(* Logix 5000 AddOnInstructionDefinition export Banner_QCM50_Param_v4; software revision 33.00; part 2 of 2 *)
(* tags used below, declared in another part *)
   QCM50 : Banner_QCM50_v4;
   Port_Data : Banner_IOL_Port_v4;
   Port : INT;   // Enter the Port number that this AOI is to work with.
   K : SINT;   // 1,3,or 5. Based off number after the K in part number.
   Local_Control : DINT;
   Command_Being_Processed : BOOL;
   Update_Archive : BOOL;
   Index_Write_Inprocess : DINT;
   Index_Write_Control : DINT;
   Inprocess_Index : DINT;
   CWC3_Index : SINT;
   CWC2_Index : SINT;
   CWC1_Index : SINT;
   C_Limit : SINT[2];
   CW_Index : SINT;
(* Banner_QCM50_Param_v4, continued *)

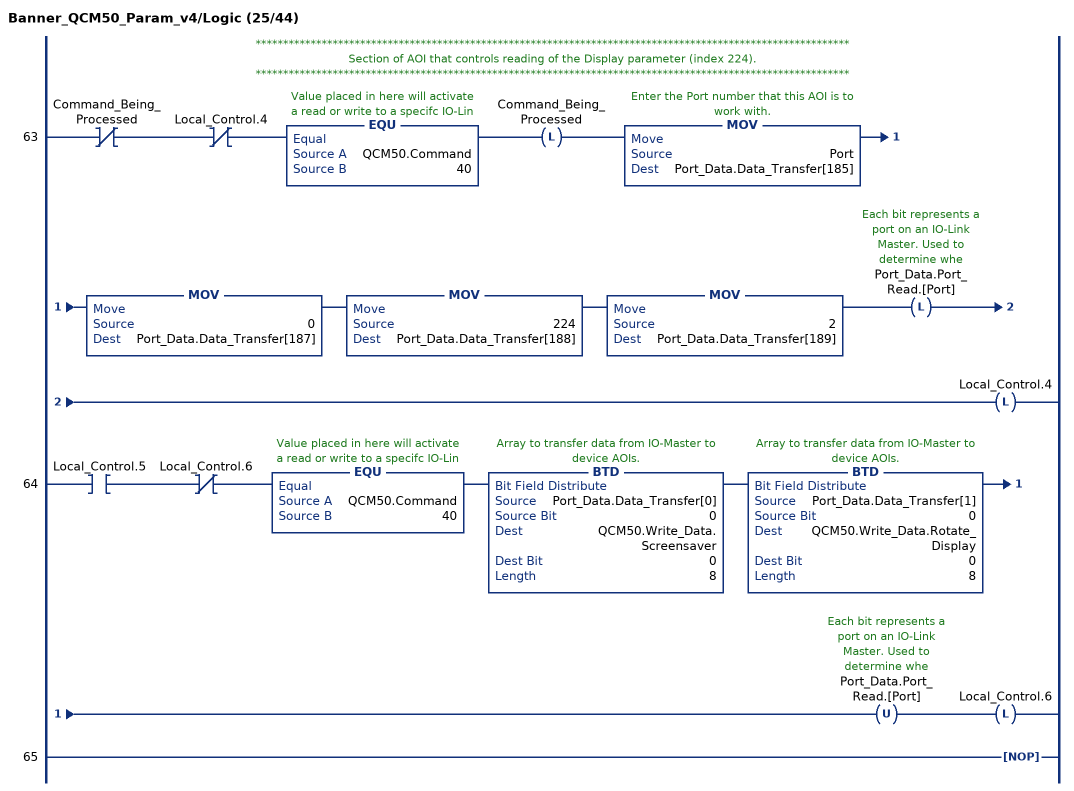
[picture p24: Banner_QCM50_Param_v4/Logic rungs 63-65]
   // ************************************************************************************************************
   // Section of AOI that controls reading of the Display parameter (index 224).
   // ************************************************************************************************************
   63: XIO(Command_Being_Processed)XIO(Local_Control.4)EQU(QCM50.Command,40)OTL(Command_Being_Processed)MOV(Port,Port_Data.Data_Transfer[185])MOV(0,Port_Data.Data_Transfer[187])MOV(224,Port_Data.Data_Transfer[188])MOV(2,Port_Data.Data_Transfer[189])OTL(Port_Data.Port_Read.[Port])OTL(Local_Control.4);
   64: XIC(Local_Control.5)XIO(Local_Control.6)EQU(QCM50.Command,40)BTD(Port_Data.Data_Transfer[0],0,QCM50.Write_Data.Screensaver,0,8)BTD(Port_Data.Data_Transfer[1],0,QCM50.Write_Data.Rotate_Display,0,8)OTU(Port_Data.Port_Read.[Port])OTL(Local_Control.6);
   65: NOP();
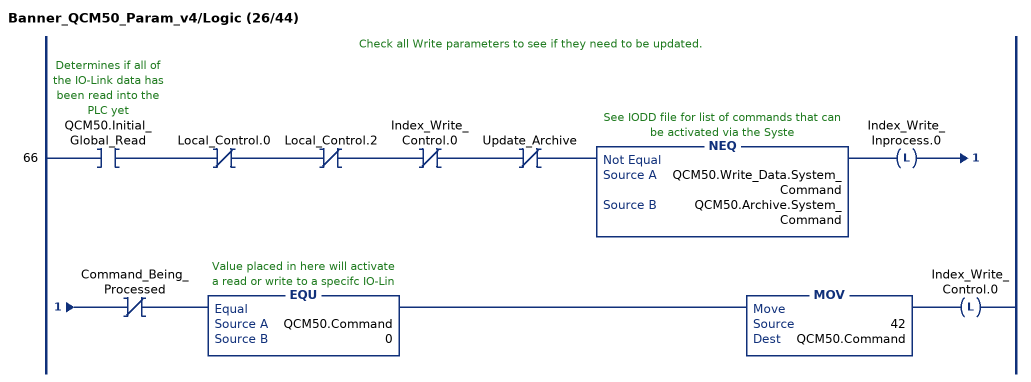
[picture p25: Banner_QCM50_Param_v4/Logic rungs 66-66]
   // Check all Write parameters to see if they need to be updated.
   66: XIC(QCM50.Initial_Global_Read)XIO(Local_Control.0)XIO(Local_Control.2)XIO(Index_Write_Control.0)XIO(Update_Archive)NEQ(QCM50.Write_Data.System_Command,QCM50.Archive.System_Command)OTL(Index_Write_Inprocess.0)XIO(Command_Being_Processed)EQU(QCM50.Command,0)MOV(42,QCM50.Command)OTL(Index_Write_Control.0);
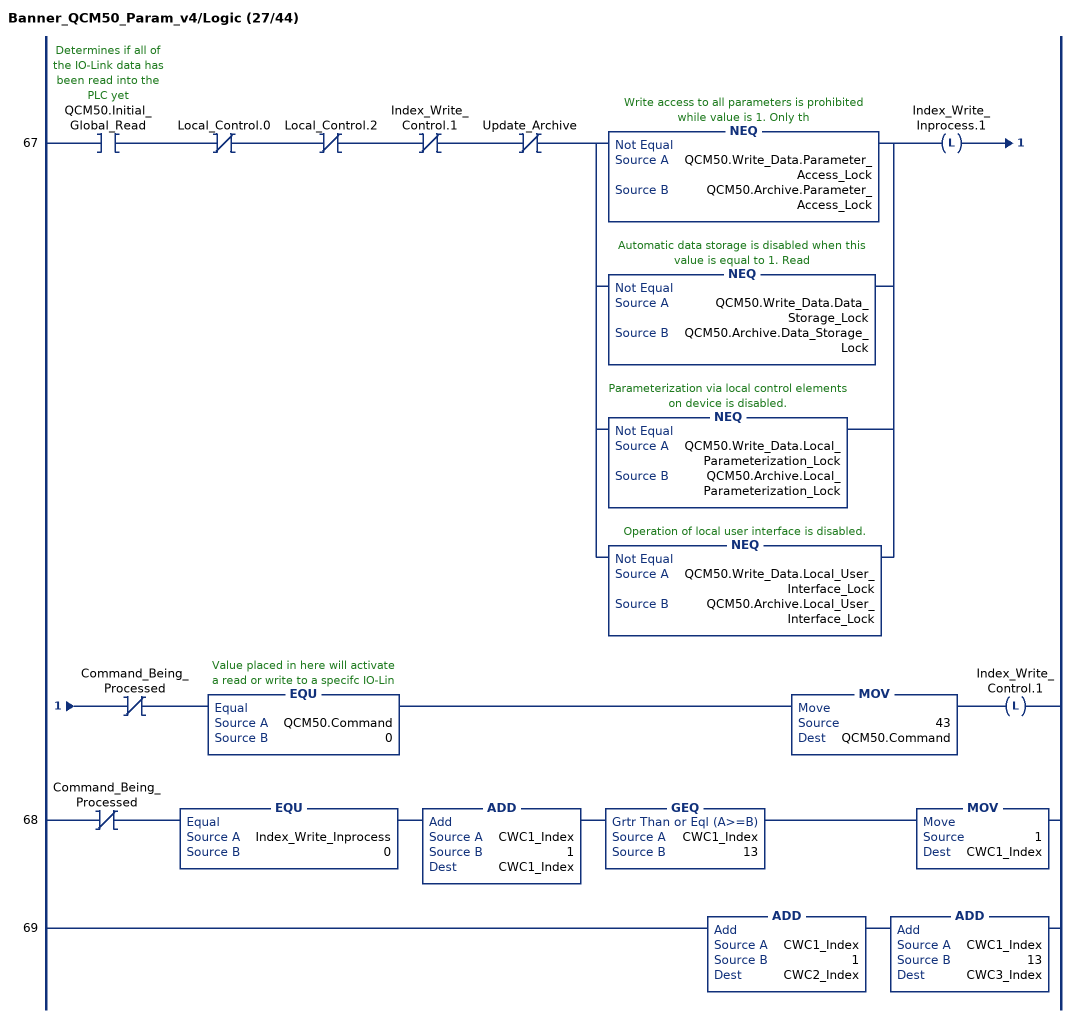
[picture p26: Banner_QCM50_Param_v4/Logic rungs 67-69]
   67: XIC(QCM50.Initial_Global_Read)XIO(Local_Control.0)XIO(Local_Control.2)XIO(Index_Write_Control.1)XIO(Update_Archive)[NEQ(QCM50.Write_Data.Parameter_Access_Lock,QCM50.Archive.Parameter_Access_Lock) ,NEQ(QCM50.Write_Data.Data_Storage_Lock,QCM50.Archive.Data_Storage_Lock) ,NEQ(QCM50.Write_Data.Local_Parameterization_Lock,QCM50.Archive.Local_Parameterization_Lock) ,NEQ(QCM50.Write_Data.Local_User_Interface_Lock,QCM50.Archive.Local_User_Interface_Lock) ]OTL(Index_Write_Inprocess.1)XIO(Command_Being_Processed)EQU(QCM50.Command,0)MOV(43,QCM50.Command)OTL(Index_Write_Control.1);
   68: XIO(Command_Being_Processed)EQU(Index_Write_Inprocess,0)ADD(CWC1_Index,1,CWC1_Index)GEQ(CWC1_Index,13)MOV(1,CWC1_Index);
   69: ADD(CWC1_Index,1,CWC2_Index)ADD(CWC1_Index,13,CWC3_Index);
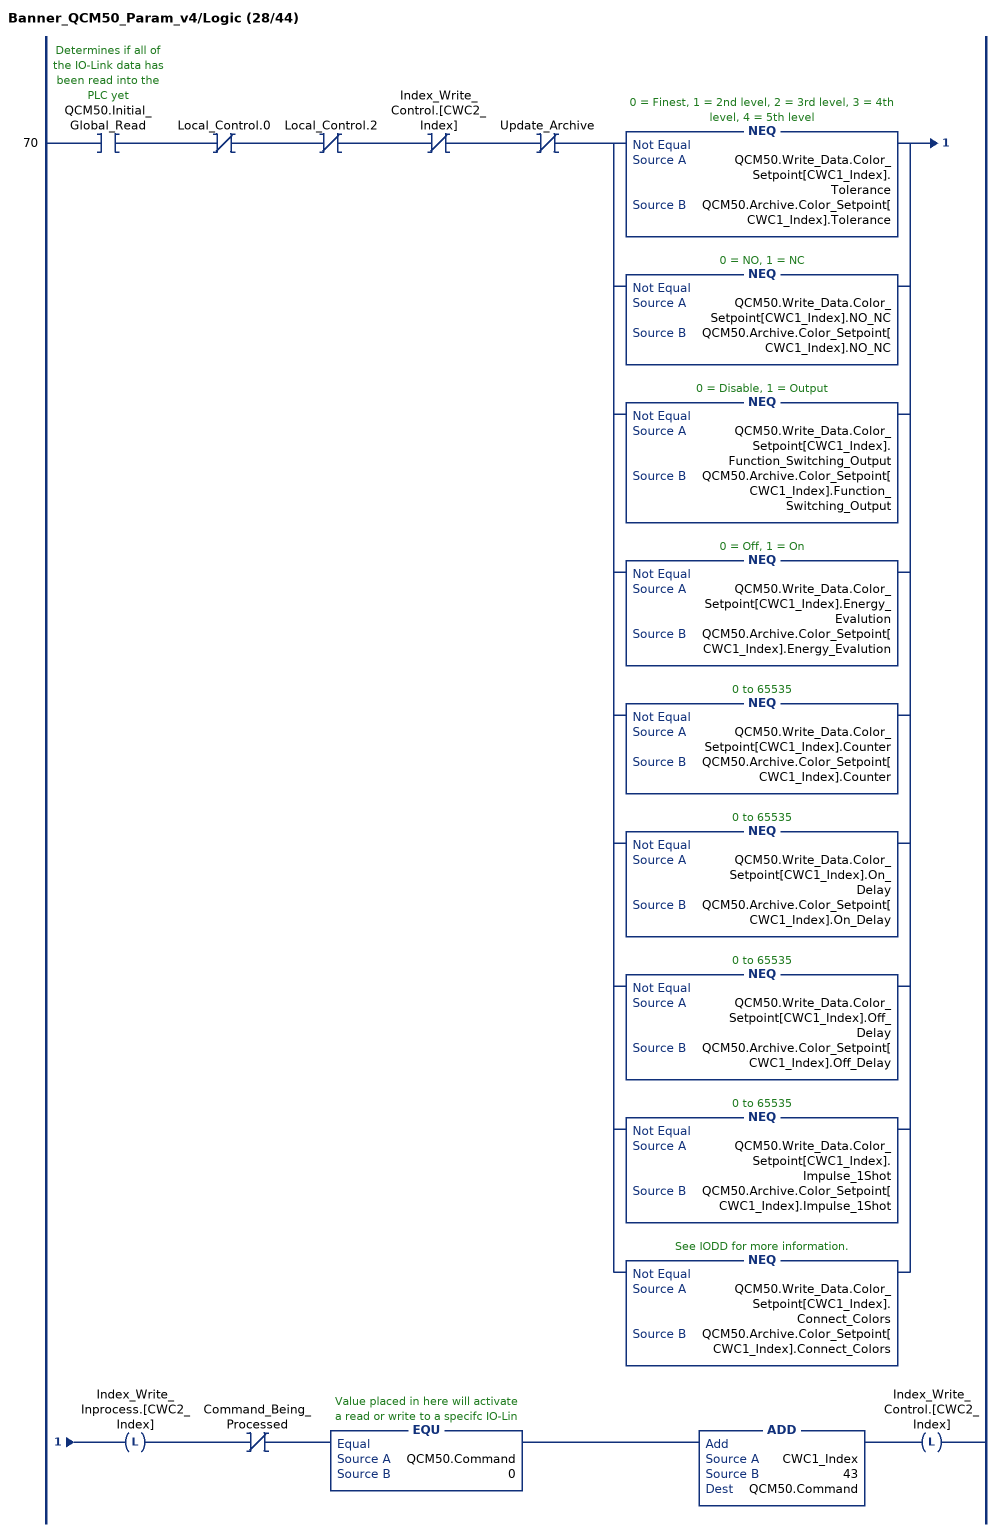
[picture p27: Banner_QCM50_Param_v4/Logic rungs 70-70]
   70: XIC(QCM50.Initial_Global_Read)XIO(Local_Control.0)XIO(Local_Control.2)XIO(Index_Write_Control.[CWC2_Index])XIO(Update_Archive)[NEQ(QCM50.Write_Data.Color_Setpoint[CWC1_Index].Tolerance,QCM50.Archive.Color_Setpoint[CWC1_Index].Tolerance) ,NEQ(QCM50.Write_Data.Color_Setpoint[CWC1_Index].NO_NC,QCM50.Archive.Color_Setpoint[CWC1_Index].NO_NC) ,NEQ(QCM50.Write_Data.Color_Setpoint[CWC1_Index].Function_Switching_Output,QCM50.Archive.Color_Setpoint[CWC1_Index].Function_Switching_Output) ,NEQ(QCM50.Write_Data.Color_Setpoint[CWC1_Index].Energy_Evalution,QCM50.Archive.Color_Setpoint[CWC1_Index].Energy_Evalution) ,NEQ(QCM50.Write_Data.Color_Setpoint[CWC1_Index].Counter,QCM50.Archive.Color_Setpoint[CWC1_Index].Counter) ,NEQ(QCM50.Write_Data.Color_Setpoint[CWC1_Index].On_Delay,QCM50.Archive.Color_Setpoint[CWC1_Index].On_Delay) ,NEQ(QCM50.Write_Data.Color_Setpoint[CWC1_Index].Off_Delay,QCM50.Archive.Color_Setpoint[CWC1_Index].Off_Delay) ,NEQ(QCM50.Write_Data.Color_Setpoint[CWC1_Index].Impulse_1Shot,QCM50.Archive.Color_Setpoint[CWC1_Index].Impulse_1Shot) ,NEQ(QCM50.Write_Data.Color_Setpoint[CWC1_Index].Connect_Colors,QCM50.Archive.Color_Setpoint[CWC1_Index].Connect_Colors) ]OTL(Index_Write_Inprocess.[CWC2_Index])XIO(Command_Being_Processed)EQU(QCM50.Command,0)ADD(CWC1_Index,43,QCM50.Command)OTL(Index_Write_Control.[CWC2_Index]);
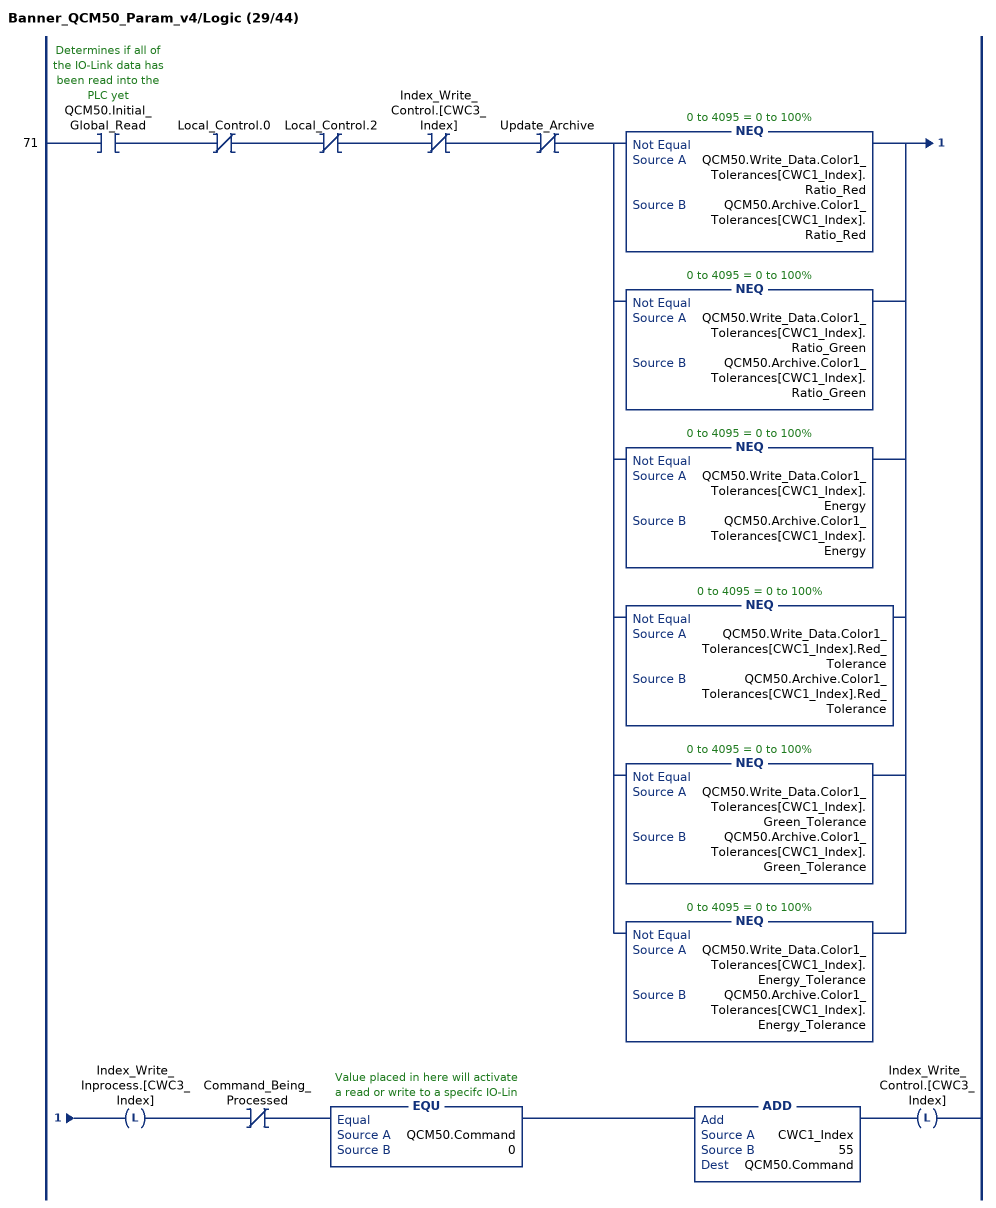
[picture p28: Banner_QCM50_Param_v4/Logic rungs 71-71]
   71: XIC(QCM50.Initial_Global_Read)XIO(Local_Control.0)XIO(Local_Control.2)XIO(Index_Write_Control.[CWC3_Index])XIO(Update_Archive)[NEQ(QCM50.Write_Data.Color1_Tolerances[CWC1_Index].Ratio_Red,QCM50.Archive.Color1_Tolerances[CWC1_Index].Ratio_Red) ,NEQ(QCM50.Write_Data.Color1_Tolerances[CWC1_Index].Ratio_Green,QCM50.Archive.Color1_Tolerances[CWC1_Index].Ratio_Green) ,NEQ(QCM50.Write_Data.Color1_Tolerances[CWC1_Index].Energy,QCM50.Archive.Color1_Tolerances[CWC1_Index].Energy) ,NEQ(QCM50.Write_Data.Color1_Tolerances[CWC1_Index].Red_Tolerance,QCM50.Archive.Color1_Tolerances[CWC1_Index].Red_Tolerance) ,NEQ(QCM50.Write_Data.Color1_Tolerances[CWC1_Index].Green_Tolerance,QCM50.Archive.Color1_Tolerances[CWC1_Index].Green_Tolerance) ,NEQ(QCM50.Write_Data.Color1_Tolerances[CWC1_Index].Energy_Tolerance,QCM50.Archive.Color1_Tolerances[CWC1_Index].Energy_Tolerance) ]OTL(Index_Write_Inprocess.[CWC3_Index])XIO(Command_Being_Processed)EQU(QCM50.Command,0)ADD(CWC1_Index,55,QCM50.Command)OTL(Index_Write_Control.[CWC3_Index]);
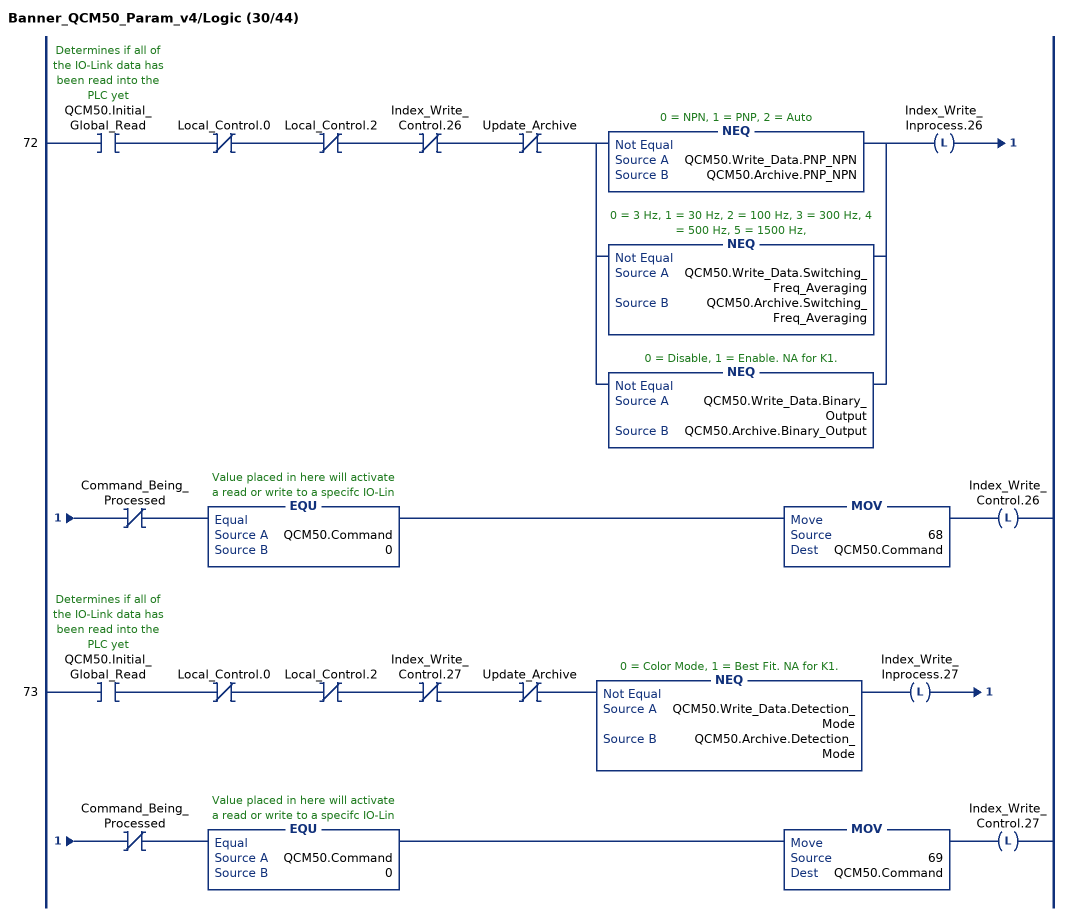
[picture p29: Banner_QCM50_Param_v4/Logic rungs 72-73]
   72: XIC(QCM50.Initial_Global_Read)XIO(Local_Control.0)XIO(Local_Control.2)XIO(Index_Write_Control.26)XIO(Update_Archive)[NEQ(QCM50.Write_Data.PNP_NPN,QCM50.Archive.PNP_NPN) ,NEQ(QCM50.Write_Data.Switching_Freq_Averaging,QCM50.Archive.Switching_Freq_Averaging) ,NEQ(QCM50.Write_Data.Binary_Output,QCM50.Archive.Binary_Output) ]OTL(Index_Write_Inprocess.26)XIO(Command_Being_Processed)EQU(QCM50.Command,0)MOV(68,QCM50.Command)OTL(Index_Write_Control.26);
   73: XIC(QCM50.Initial_Global_Read)XIO(Local_Control.0)XIO(Local_Control.2)XIO(Index_Write_Control.27)XIO(Update_Archive)NEQ(QCM50.Write_Data.Detection_Mode,QCM50.Archive.Detection_Mode)OTL(Index_Write_Inprocess.27)XIO(Command_Being_Processed)EQU(QCM50.Command,0)MOV(69,QCM50.Command)OTL(Index_Write_Control.27);
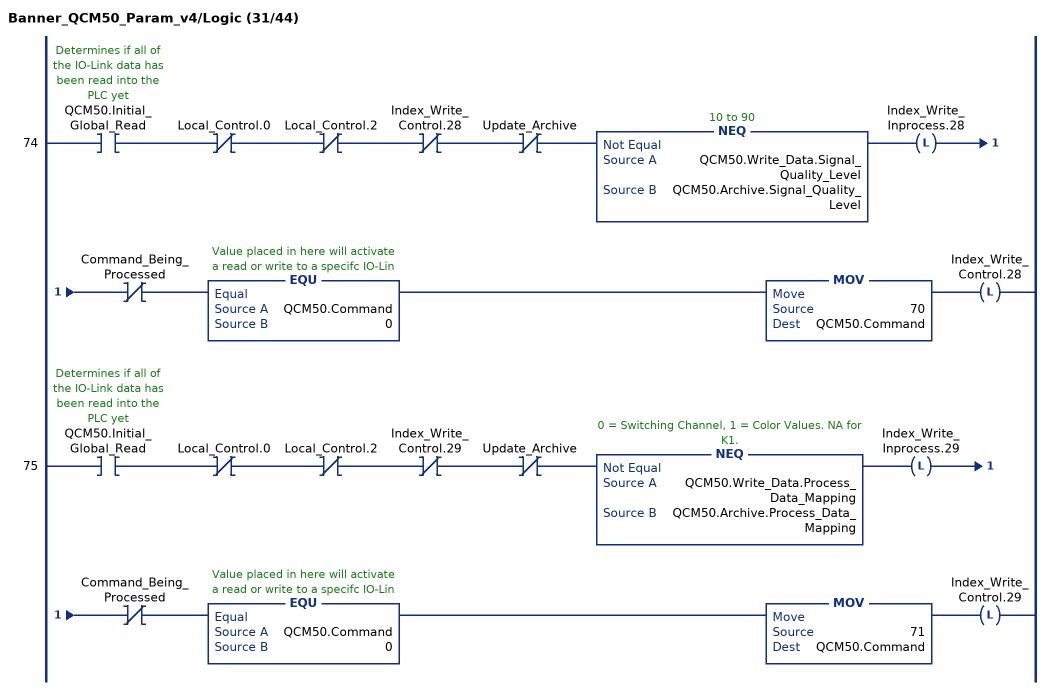
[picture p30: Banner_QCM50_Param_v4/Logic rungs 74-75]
   74: XIC(QCM50.Initial_Global_Read)XIO(Local_Control.0)XIO(Local_Control.2)XIO(Index_Write_Control.28)XIO(Update_Archive)NEQ(QCM50.Write_Data.Signal_Quality_Level,QCM50.Archive.Signal_Quality_Level)OTL(Index_Write_Inprocess.28)XIO(Command_Being_Processed)EQU(QCM50.Command,0)MOV(70,QCM50.Command)OTL(Index_Write_Control.28);
   75: XIC(QCM50.Initial_Global_Read)XIO(Local_Control.0)XIO(Local_Control.2)XIO(Index_Write_Control.29)XIO(Update_Archive)NEQ(QCM50.Write_Data.Process_Data_Mapping,QCM50.Archive.Process_Data_Mapping)OTL(Index_Write_Inprocess.29)XIO(Command_Being_Processed)EQU(QCM50.Command,0)MOV(71,QCM50.Command)OTL(Index_Write_Control.29);
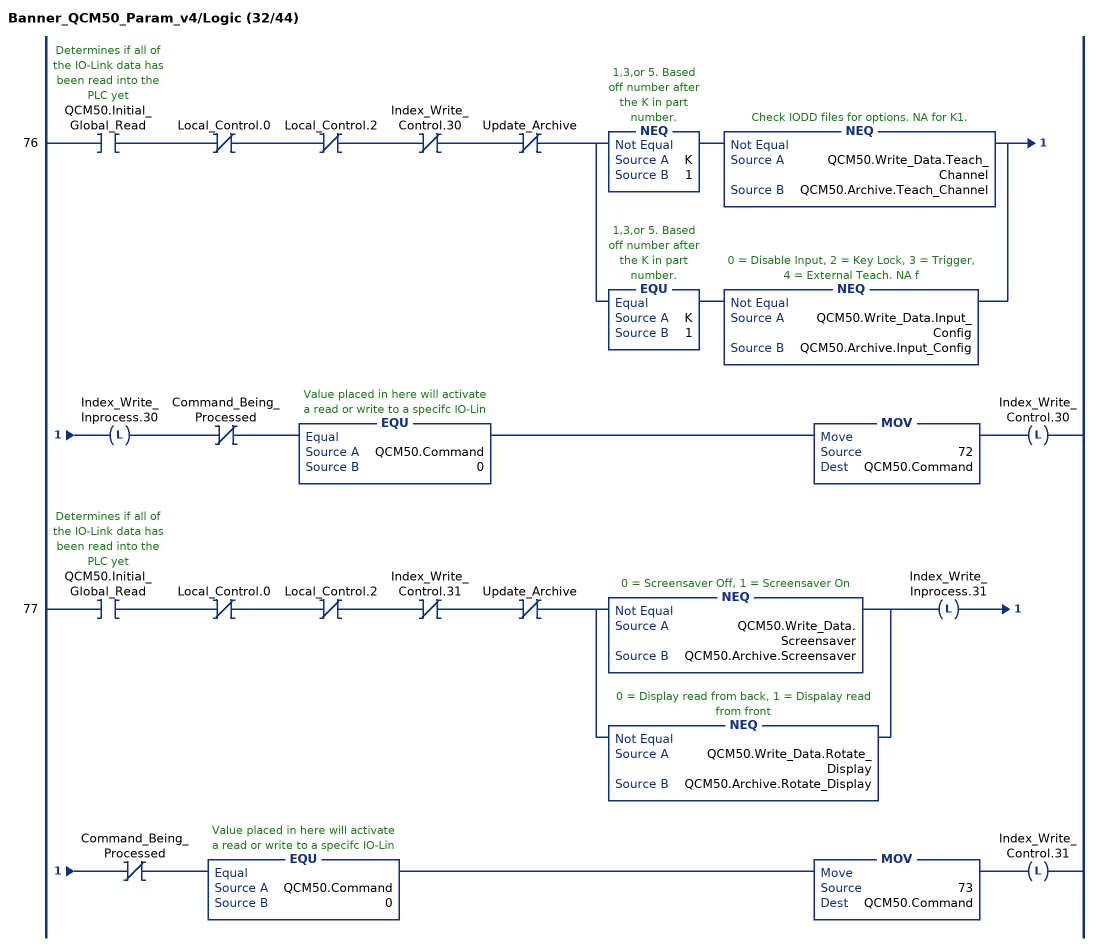
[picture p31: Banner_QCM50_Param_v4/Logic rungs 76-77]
   76: XIC(QCM50.Initial_Global_Read)XIO(Local_Control.0)XIO(Local_Control.2)XIO(Index_Write_Control.30)XIO(Update_Archive)[NEQ(K,1) NEQ(QCM50.Write_Data.Teach_Channel,QCM50.Archive.Teach_Channel) ,EQU(K,1) NEQ(QCM50.Write_Data.Input_Config,QCM50.Archive.Input_Config) ]OTL(Index_Write_Inprocess.30)XIO(Command_Being_Processed)EQU(QCM50.Command,0)MOV(72,QCM50.Command)OTL(Index_Write_Control.30);
   77: XIC(QCM50.Initial_Global_Read)XIO(Local_Control.0)XIO(Local_Control.2)XIO(Index_Write_Control.31)XIO(Update_Archive)[NEQ(QCM50.Write_Data.Screensaver,QCM50.Archive.Screensaver) ,NEQ(QCM50.Write_Data.Rotate_Display,QCM50.Archive.Rotate_Display) ]OTL(Index_Write_Inprocess.31)XIO(Command_Being_Processed)EQU(QCM50.Command,0)MOV(73,QCM50.Command)OTL(Index_Write_Control.31);
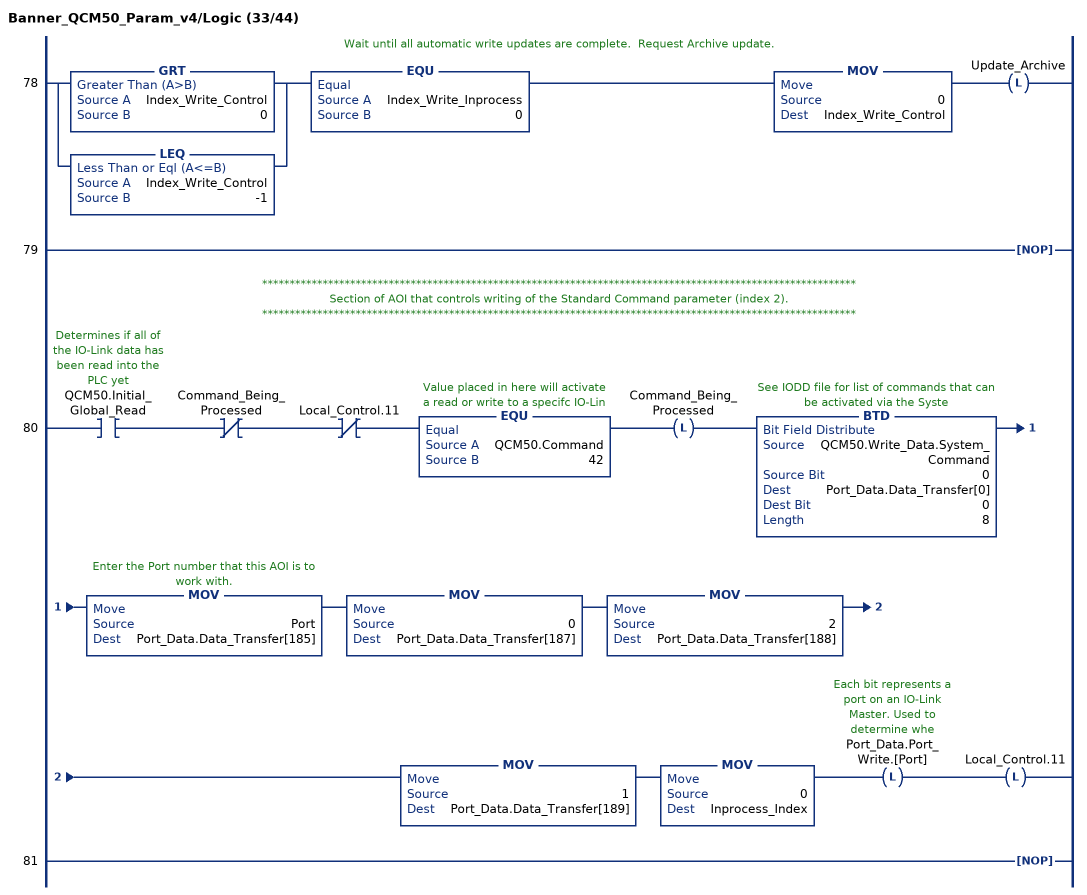
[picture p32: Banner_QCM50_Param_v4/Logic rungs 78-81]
   // Wait until all automatic write updates are complete.  Request Archive update.
   78: [GRT(Index_Write_Control,0) ,LEQ(Index_Write_Control,-1) ]EQU(Index_Write_Inprocess,0)MOV(0,Index_Write_Control)OTL(Update_Archive);
   79: NOP();
   // ************************************************************************************************************
   // Section of AOI that controls writing of the Standard Command parameter (index 2).
   // ************************************************************************************************************
   80: XIC(QCM50.Initial_Global_Read)XIO(Command_Being_Processed)XIO(Local_Control.11)EQU(QCM50.Command,42)OTL(Command_Being_Processed)BTD(QCM50.Write_Data.System_Command,0,Port_Data.Data_Transfer[0],0,8)MOV(Port,Port_Data.Data_Transfer[185])MOV(0,Port_Data.Data_Transfer[187])MOV(2,Port_Data.Data_Transfer[188])MOV(1,Port_Data.Data_Transfer[189])MOV(0,Inprocess_Index)OTL(Port_Data.Port_Write.[Port])OTL(Local_Control.11);
   81: NOP();
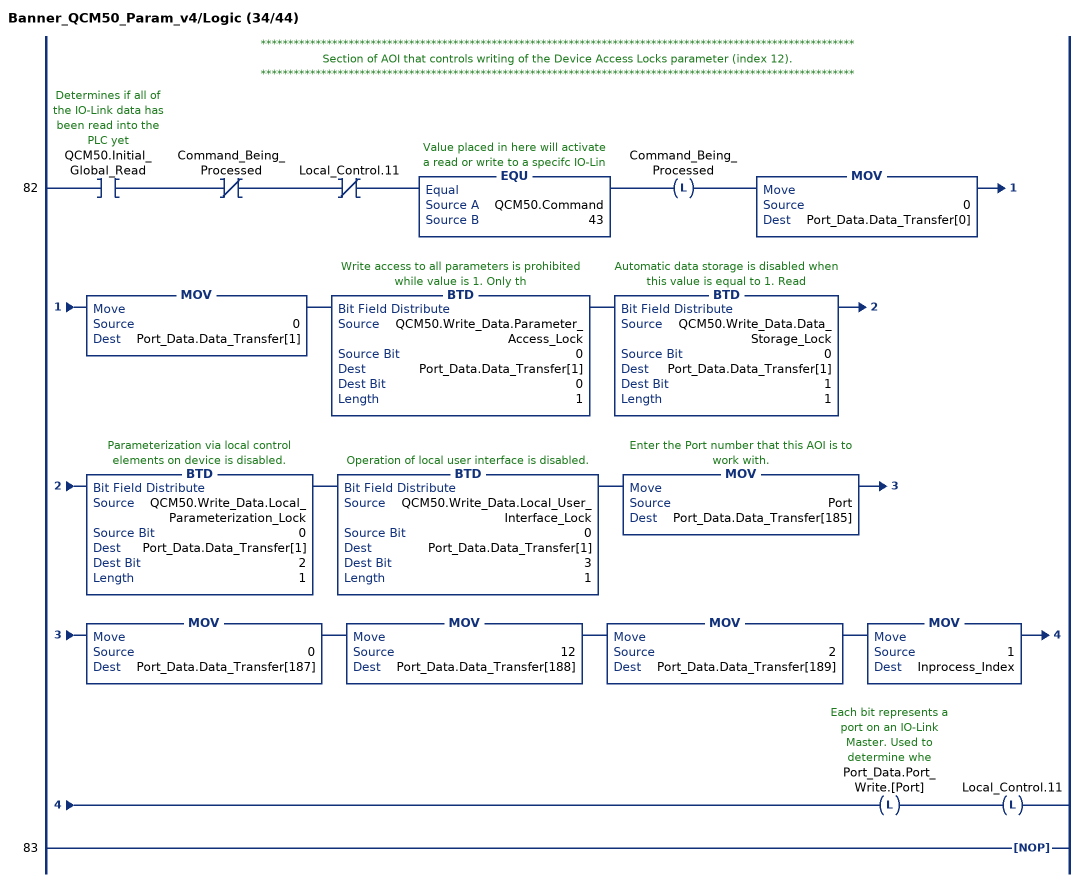
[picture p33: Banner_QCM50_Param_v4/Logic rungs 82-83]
   // ************************************************************************************************************
   // Section of AOI that controls writing of the Device Access Locks parameter (index 12).
   // ************************************************************************************************************
   82: XIC(QCM50.Initial_Global_Read)XIO(Command_Being_Processed)XIO(Local_Control.11)EQU(QCM50.Command,43)OTL(Command_Being_Processed)MOV(0,Port_Data.Data_Transfer[0])MOV(0,Port_Data.Data_Transfer[1])BTD(QCM50.Write_Data.Parameter_Access_Lock,0,Port_Data.Data_Transfer[1],0,1)BTD(QCM50.Write_Data.Data_Storage_Lock,0,Port_Data.Data_Transfer[1],1,1)BTD(QCM50.Write_Data.Local_Parameterization_Lock,0,Port_Data.Data_Transfer[1],2,1)BTD(QCM50.Write_Data.Local_User_Interface_Lock,0,Port_Data.Data_Transfer[1],3,1)MOV(Port,Port_Data.Data_Transfer[185])MOV(0,Port_Data.Data_Transfer[187])MOV(12,Port_Data.Data_Transfer[188])MOV(2,Port_Data.Data_Transfer[189])MOV(1,Inprocess_Index)OTL(Port_Data.Port_Write.[Port])OTL(Local_Control.11);
   83: NOP();
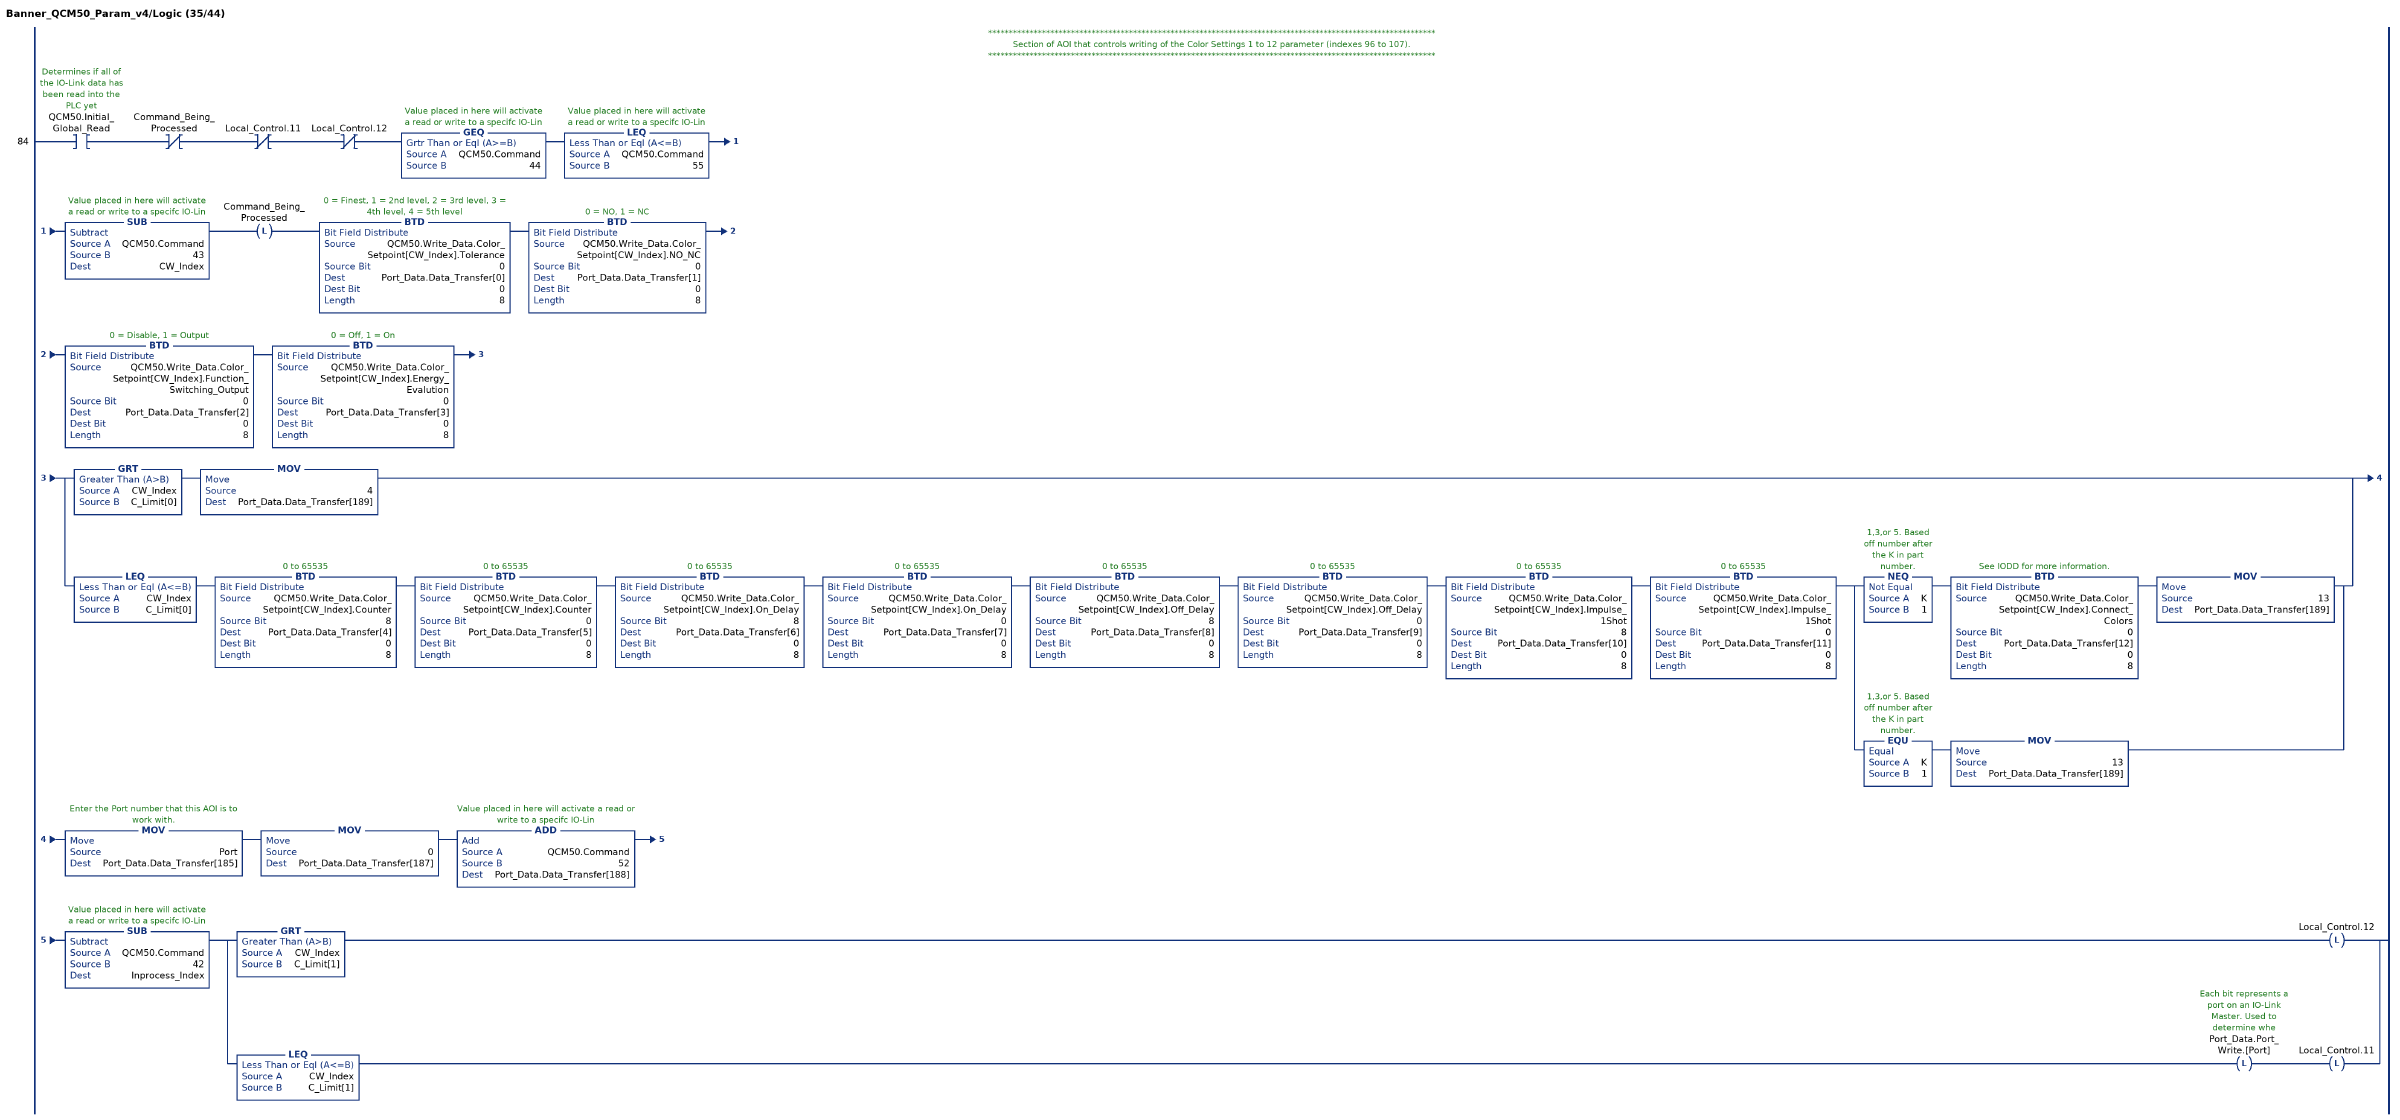
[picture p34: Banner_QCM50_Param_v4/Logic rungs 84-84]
   // ************************************************************************************************************
   // Section of AOI that controls writing of the Color Settings 1 to 12 parameter (indexes 96 to 107).
   // ************************************************************************************************************
   84: XIC(QCM50.Initial_Global_Read)XIO(Command_Being_Processed)XIO(Local_Control.11)XIO(Local_Control.12)GEQ(QCM50.Command,44)LEQ(QCM50.Command,55)SUB(QCM50.Command,43,CW_Index)OTL(Command_Being_Processed)BTD(QCM50.Write_Data.Color_Setpoint[CW_Index].Tolerance,0,Port_Data.Data_Transfer[0],0,8)BTD(QCM50.Write_Data.Color_Setpoint[CW_Index].NO_NC,0,Port_Data.Data_Transfer[1],0,8)BTD(QCM50.Write_Data.Color_Setpoint[CW_Index].Function_Switching_Output,0,Port_Data.Data_Transfer[2],0,8)BTD(QCM50.Write_Data.Color_Setpoint[CW_Index].Energy_Evalution,0,Port_Data.Data_Transfer[3],0,8)[GRT(CW_Index,C_Limit[0]) MOV(4,Port_Data.Data_Transfer[189]) ,LEQ(CW_Index,C_Limit[0]) BTD(QCM50.Write_Data.Color_Setpoint[CW_Index].Counter,8,Port_Data.Data_Transfer[4],0,8) BTD(QCM50.Write_Data.Color_Setpoint[CW_Index].Counter,0,Port_Data.Data_Transfer[5],0,8) BTD(QCM50.Write_Data.Color_Setpoint[CW_Index].On_Delay,8,Port_Data.Data_Transfer[6],0,8) BTD(QCM50.Write_Data.Color_Setpoint[CW_Index].On_Delay,0,Port_Data.Data_Transfer[7],0,8) BTD(QCM50.Write_Data.Color_Setpoint[CW_Index].Off_Delay,8,Port_Data.Data_Transfer[8],0,8) BTD(QCM50.Write_Data.Color_Setpoint[CW_Index].Off_Delay,0,Port_Data.Data_Transfer[9],0,8) BTD(QCM50.Write_Data.Color_Setpoint[CW_Index].Impulse_1Shot,8,Port_Data.Data_Transfer[10],0,8) BTD(QCM50.Write_Data.Color_Setpoint[CW_Index].Impulse_1Shot,0,Port_Data.Data_Transfer[11],0,8) [NEQ(K,1) BTD(QCM50.Write_Data.Color_Setpoint[CW_Index].Connect_Colors,0,Port_Data.Data_Transfer[12],0,8) MOV(13,Port_Data.Data_Transfer[189]) ,EQU(K,1) MOV(13,Port_Data.Data_Transfer[189]) ] ]MOV(Port,Port_Data.Data_Transfer[185])MOV(0,Port_Data.Data_Transfer[187])ADD(QCM50.Command,52,Port_Data.Data_Transfer[188])SUB(QCM50.Command,42,Inprocess_Index)[GRT(CW_Index,C_Limit[1]) OTL(Local_Control.12) ,LEQ(CW_Index,C_Limit[1]) OTL(Port_Data.Port_Write.[Port]) OTL(Local_Control.11) ];
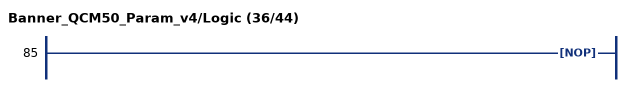
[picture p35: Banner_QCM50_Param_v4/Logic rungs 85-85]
   85: NOP();
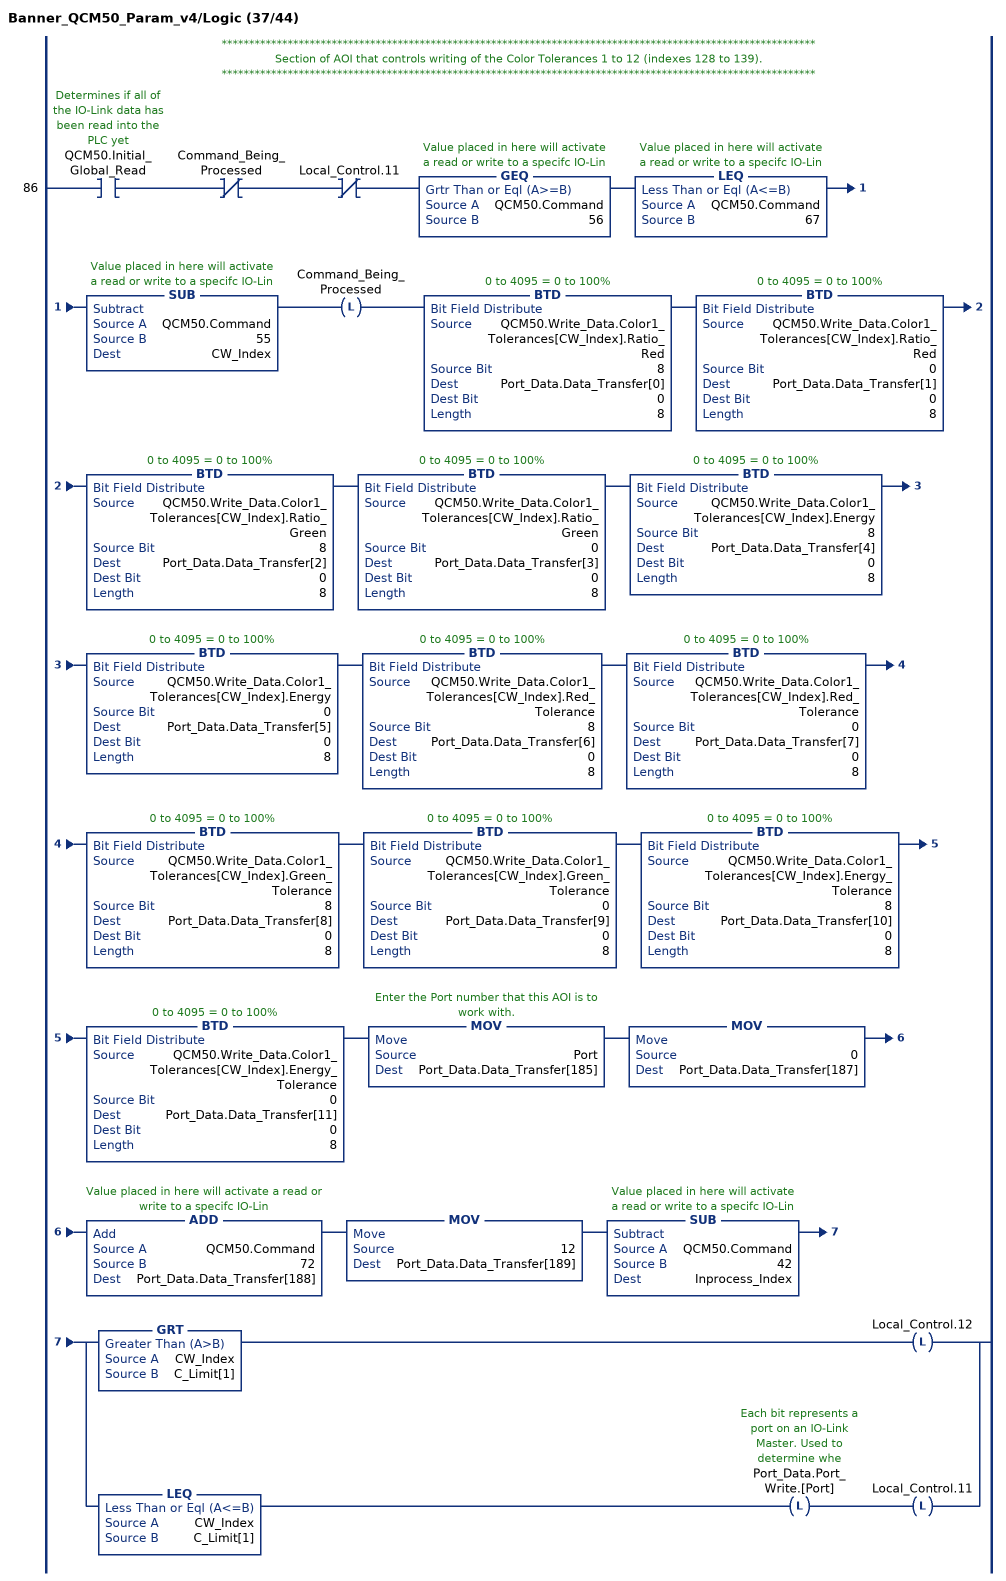
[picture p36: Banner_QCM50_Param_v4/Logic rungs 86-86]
   // ************************************************************************************************************
   // Section of AOI that controls writing of the Color Tolerances 1 to 12 (indexes 128 to 139).
   // ************************************************************************************************************
   86: XIC(QCM50.Initial_Global_Read)XIO(Command_Being_Processed)XIO(Local_Control.11)GEQ(QCM50.Command,56)LEQ(QCM50.Command,67)SUB(QCM50.Command,55,CW_Index)OTL(Command_Being_Processed)BTD(QCM50.Write_Data.Color1_Tolerances[CW_Index].Ratio_Red,8,Port_Data.Data_Transfer[0],0,8)BTD(QCM50.Write_Data.Color1_Tolerances[CW_Index].Ratio_Red,0,Port_Data.Data_Transfer[1],0,8)BTD(QCM50.Write_Data.Color1_Tolerances[CW_Index].Ratio_Green,8,Port_Data.Data_Transfer[2],0,8)BTD(QCM50.Write_Data.Color1_Tolerances[CW_Index].Ratio_Green,0,Port_Data.Data_Transfer[3],0,8)BTD(QCM50.Write_Data.Color1_Tolerances[CW_Index].Energy,8,Port_Data.Data_Transfer[4],0,8)BTD(QCM50.Write_Data.Color1_Tolerances[CW_Index].Energy,0,Port_Data.Data_Transfer[5],0,8)BTD(QCM50.Write_Data.Color1_Tolerances[CW_Index].Red_Tolerance,8,Port_Data.Data_Transfer[6],0,8)BTD(QCM50.Write_Data.Color1_Tolerances[CW_Index].Red_Tolerance,0,Port_Data.Data_Transfer[7],0,8)BTD(QCM50.Write_Data.Color1_Tolerances[CW_Index].Green_Tolerance,8,Port_Data.Data_Transfer[8],0,8)BTD(QCM50.Write_Data.Color1_Tolerances[CW_Index].Green_Tolerance,0,Port_Data.Data_Transfer[9],0,8)BTD(QCM50.Write_Data.Color1_Tolerances[CW_Index].Energy_Tolerance,8,Port_Data.Data_Transfer[10],0,8)BTD(QCM50.Write_Data.Color1_Tolerances[CW_Index].Energy_Tolerance,0,Port_Data.Data_Transfer[11],0,8)MOV(Port,Port_Data.Data_Transfer[185])MOV(0,Port_Data.Data_Transfer[187])ADD(QCM50.Command,72,Port_Data.Data_Transfer[188])MOV(12,Port_Data.Data_Transfer[189])SUB(QCM50.Command,42,Inprocess_Index)[GRT(CW_Index,C_Limit[1]) OTL(Local_Control.12) ,LEQ(CW_Index,C_Limit[1]) OTL(Port_Data.Port_Write.[Port]) OTL(Local_Control.11) ];
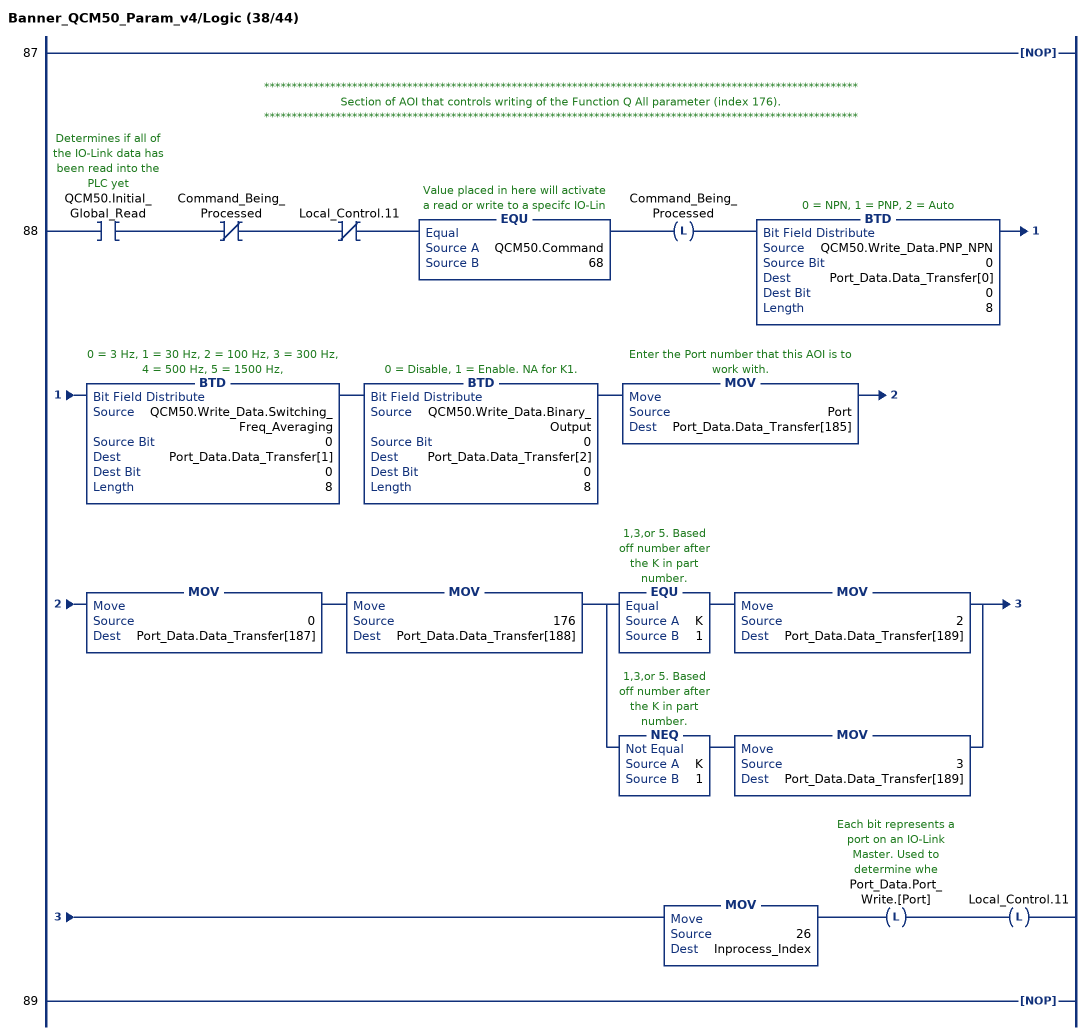
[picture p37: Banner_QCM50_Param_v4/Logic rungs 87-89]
   87: NOP();
   // ************************************************************************************************************
   // Section of AOI that controls writing of the Function Q All parameter (index 176).
   // ************************************************************************************************************
   88: XIC(QCM50.Initial_Global_Read)XIO(Command_Being_Processed)XIO(Local_Control.11)EQU(QCM50.Command,68)OTL(Command_Being_Processed)BTD(QCM50.Write_Data.PNP_NPN,0,Port_Data.Data_Transfer[0],0,8)BTD(QCM50.Write_Data.Switching_Freq_Averaging,0,Port_Data.Data_Transfer[1],0,8)BTD(QCM50.Write_Data.Binary_Output,0,Port_Data.Data_Transfer[2],0,8)MOV(Port,Port_Data.Data_Transfer[185])MOV(0,Port_Data.Data_Transfer[187])MOV(176,Port_Data.Data_Transfer[188])[EQU(K,1) MOV(2,Port_Data.Data_Transfer[189]) ,NEQ(K,1) MOV(3,Port_Data.Data_Transfer[189]) ]MOV(26,Inprocess_Index)OTL(Port_Data.Port_Write.[Port])OTL(Local_Control.11);
   89: NOP();
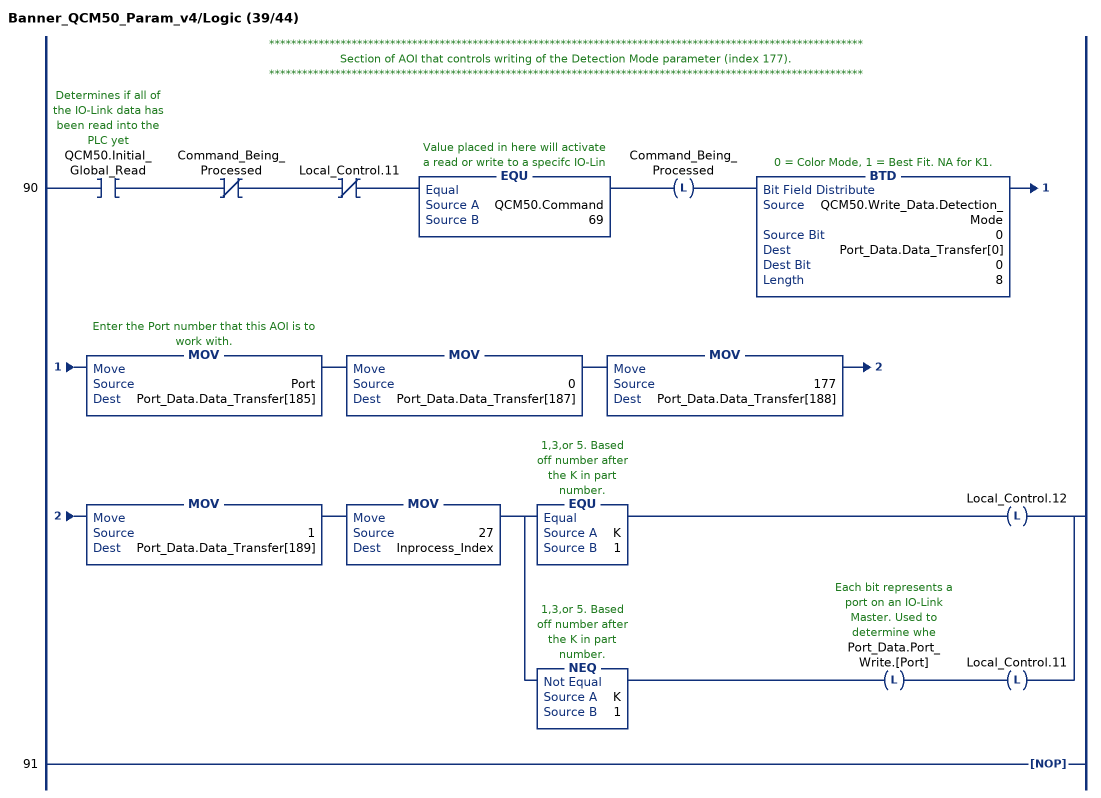
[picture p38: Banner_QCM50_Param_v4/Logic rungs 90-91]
   // ************************************************************************************************************
   // Section of AOI that controls writing of the Detection Mode parameter (index 177).
   // ************************************************************************************************************
   90: XIC(QCM50.Initial_Global_Read)XIO(Command_Being_Processed)XIO(Local_Control.11)EQU(QCM50.Command,69)OTL(Command_Being_Processed)BTD(QCM50.Write_Data.Detection_Mode,0,Port_Data.Data_Transfer[0],0,8)MOV(Port,Port_Data.Data_Transfer[185])MOV(0,Port_Data.Data_Transfer[187])MOV(177,Port_Data.Data_Transfer[188])MOV(1,Port_Data.Data_Transfer[189])MOV(27,Inprocess_Index)[EQU(K,1) OTL(Local_Control.12) ,NEQ(K,1) OTL(Port_Data.Port_Write.[Port]) OTL(Local_Control.11) ];
   91: NOP();
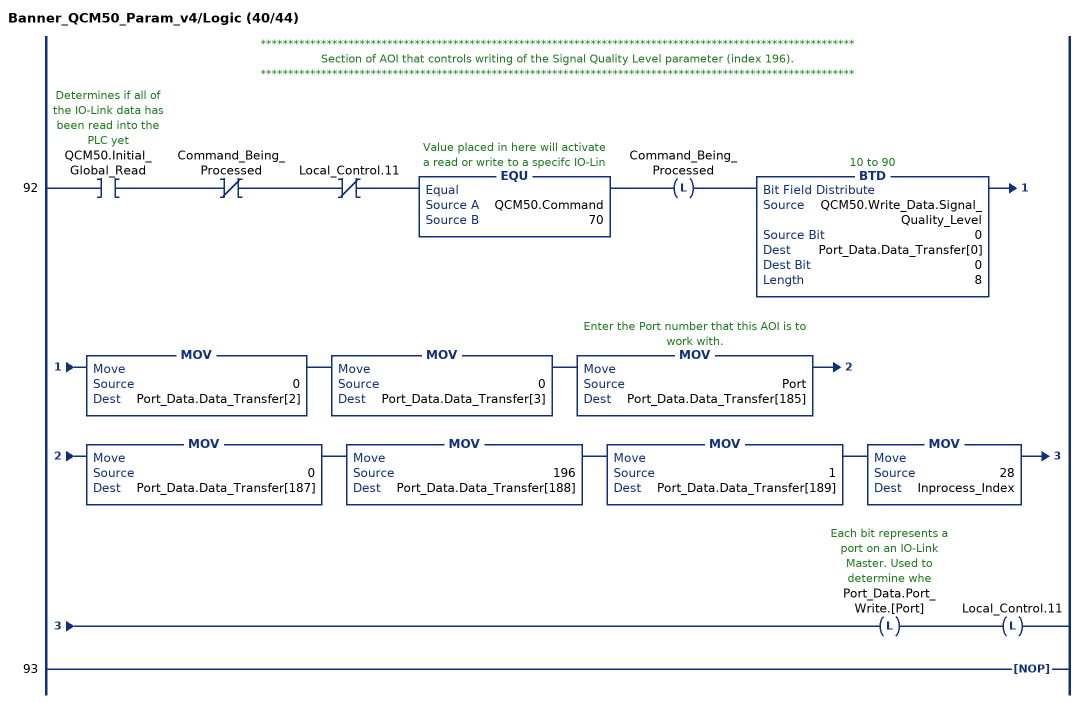
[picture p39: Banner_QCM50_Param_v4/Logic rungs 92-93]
   // ************************************************************************************************************
   // Section of AOI that controls writing of the Signal Quality Level parameter (index 196).
   // ************************************************************************************************************
   92: XIC(QCM50.Initial_Global_Read)XIO(Command_Being_Processed)XIO(Local_Control.11)EQU(QCM50.Command,70)OTL(Command_Being_Processed)BTD(QCM50.Write_Data.Signal_Quality_Level,0,Port_Data.Data_Transfer[0],0,8)MOV(0,Port_Data.Data_Transfer[2])MOV(0,Port_Data.Data_Transfer[3])MOV(Port,Port_Data.Data_Transfer[185])MOV(0,Port_Data.Data_Transfer[187])MOV(196,Port_Data.Data_Transfer[188])MOV(1,Port_Data.Data_Transfer[189])MOV(28,Inprocess_Index)OTL(Port_Data.Port_Write.[Port])OTL(Local_Control.11);
   93: NOP();
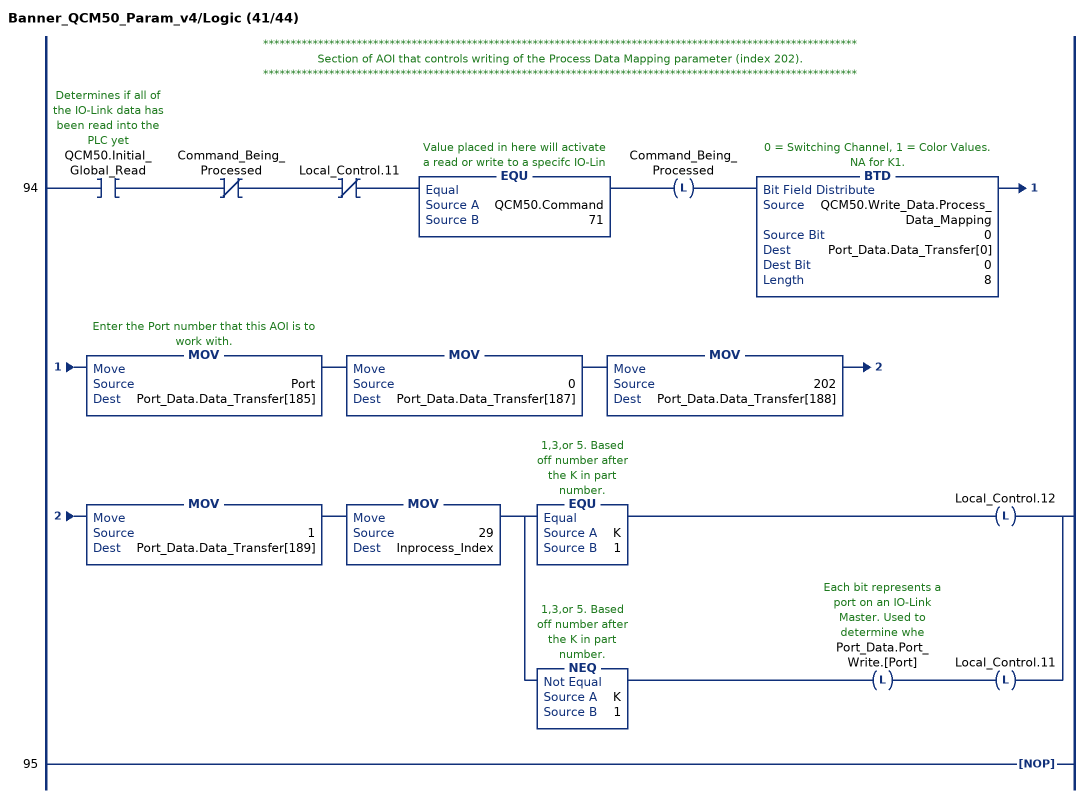
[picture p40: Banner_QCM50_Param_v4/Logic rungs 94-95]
   // ************************************************************************************************************
   // Section of AOI that controls writing of the Process Data Mapping parameter (index 202).
   // ************************************************************************************************************
   94: XIC(QCM50.Initial_Global_Read)XIO(Command_Being_Processed)XIO(Local_Control.11)EQU(QCM50.Command,71)OTL(Command_Being_Processed)BTD(QCM50.Write_Data.Process_Data_Mapping,0,Port_Data.Data_Transfer[0],0,8)MOV(Port,Port_Data.Data_Transfer[185])MOV(0,Port_Data.Data_Transfer[187])MOV(202,Port_Data.Data_Transfer[188])MOV(1,Port_Data.Data_Transfer[189])MOV(29,Inprocess_Index)[EQU(K,1) OTL(Local_Control.12) ,NEQ(K,1) OTL(Port_Data.Port_Write.[Port]) OTL(Local_Control.11) ];
   95: NOP();
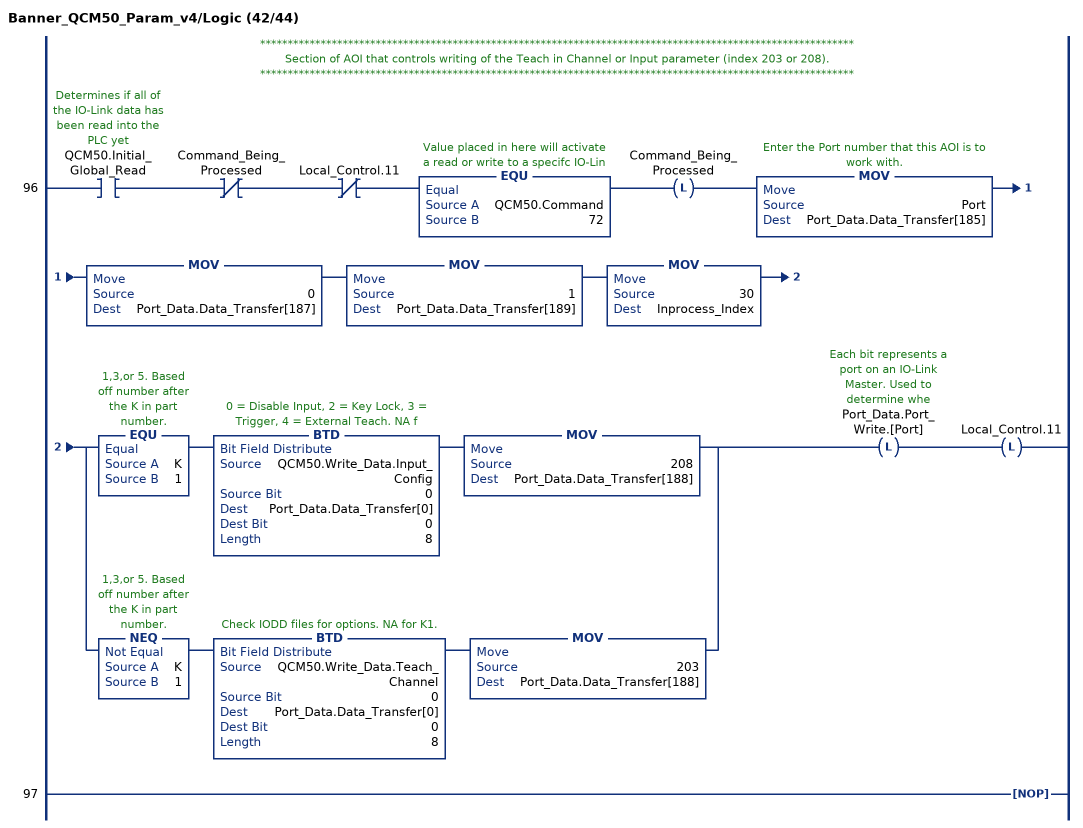
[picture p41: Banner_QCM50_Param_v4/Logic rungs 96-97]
   // ************************************************************************************************************
   // Section of AOI that controls writing of the Teach in Channel or Input parameter (index 203 or 208).
   // ************************************************************************************************************
   96: XIC(QCM50.Initial_Global_Read)XIO(Command_Being_Processed)XIO(Local_Control.11)EQU(QCM50.Command,72)OTL(Command_Being_Processed)MOV(Port,Port_Data.Data_Transfer[185])MOV(0,Port_Data.Data_Transfer[187])MOV(1,Port_Data.Data_Transfer[189])MOV(30,Inprocess_Index)[EQU(K,1) BTD(QCM50.Write_Data.Input_Config,0,Port_Data.Data_Transfer[0],0,8) MOV(208,Port_Data.Data_Transfer[188]) ,NEQ(K,1) BTD(QCM50.Write_Data.Teach_Channel,0,Port_Data.Data_Transfer[0],0,8) MOV(203,Port_Data.Data_Transfer[188]) ]OTL(Port_Data.Port_Write.[Port])OTL(Local_Control.11);
   97: NOP();
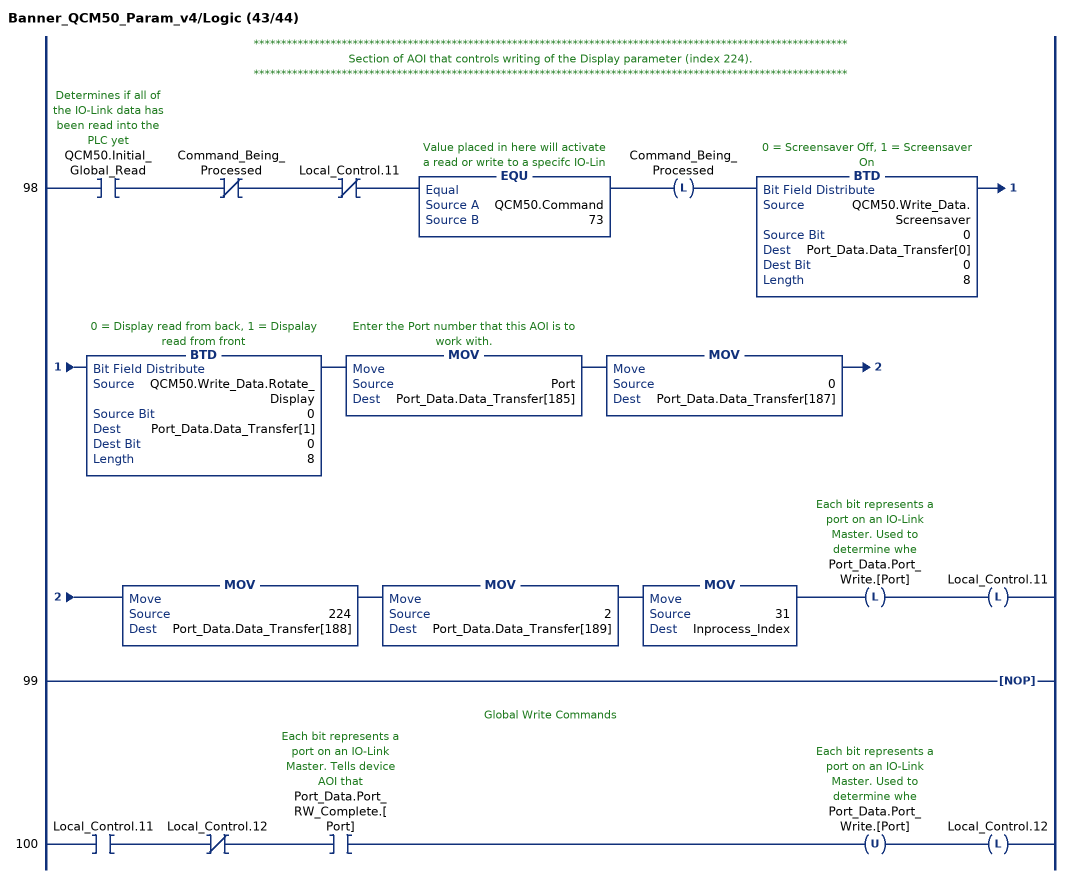
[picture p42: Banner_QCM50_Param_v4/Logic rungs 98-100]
   // ************************************************************************************************************
   // Section of AOI that controls writing of the Display parameter (index 224).
   // ************************************************************************************************************
   98: XIC(QCM50.Initial_Global_Read)XIO(Command_Being_Processed)XIO(Local_Control.11)EQU(QCM50.Command,73)OTL(Command_Being_Processed)BTD(QCM50.Write_Data.Screensaver,0,Port_Data.Data_Transfer[0],0,8)BTD(QCM50.Write_Data.Rotate_Display,0,Port_Data.Data_Transfer[1],0,8)MOV(Port,Port_Data.Data_Transfer[185])MOV(0,Port_Data.Data_Transfer[187])MOV(224,Port_Data.Data_Transfer[188])MOV(2,Port_Data.Data_Transfer[189])MOV(31,Inprocess_Index)OTL(Port_Data.Port_Write.[Port])OTL(Local_Control.11);
   99: NOP();
   // Global Write Commands
   100: XIC(Local_Control.11)XIO(Local_Control.12)XIC(Port_Data.Port_RW_Complete.[Port])OTU(Port_Data.Port_Write.[Port])OTL(Local_Control.12);
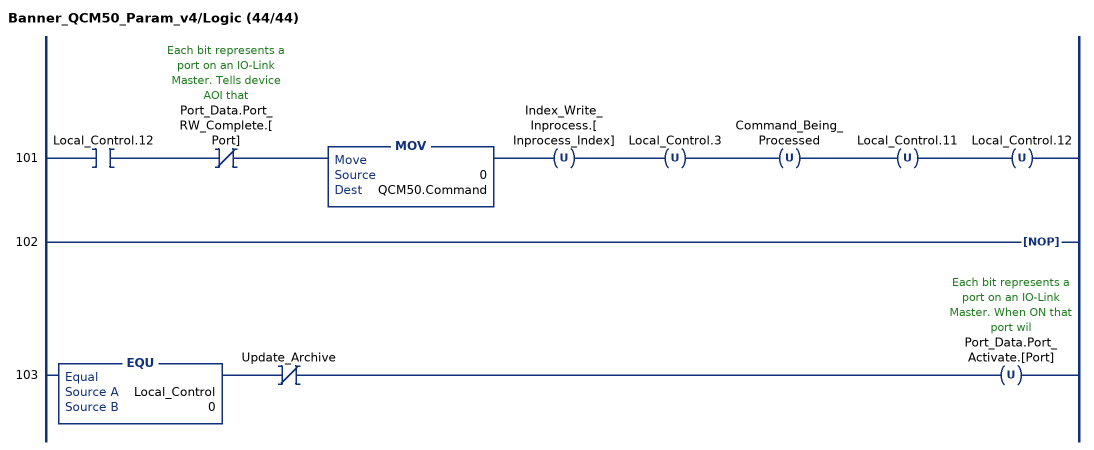
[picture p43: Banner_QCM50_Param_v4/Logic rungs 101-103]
   101: XIC(Local_Control.12)XIO(Port_Data.Port_RW_Complete.[Port])MOV(0,QCM50.Command)OTU(Index_Write_Inprocess.[Inprocess_Index])OTU(Local_Control.3)OTU(Command_Being_Processed)OTU(Local_Control.11)OTU(Local_Control.12);
   102: NOP();
   103: EQU(Local_Control,0)XIO(Update_Archive)OTU(Port_Data.Port_Activate.[Port]);
END_ROUTINE
END_ADD_ON_INSTRUCTION
